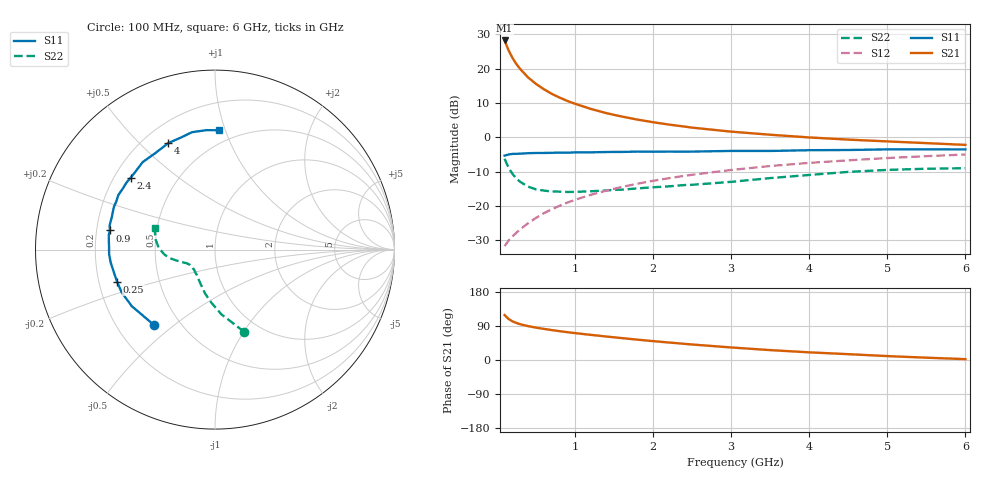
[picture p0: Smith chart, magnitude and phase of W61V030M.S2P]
! SIEMENS Small Signal Semiconductors
! BFR193W
! Si NPN RF Bipolar Junction Transistor in SOT323
! VCE = 1 V  IC = 30 mA
! Common Emitter S-Parameters:  September  1992
# GHz  S  MA  R  50
!  f  S11  S21  S12  S22
! GHz  MAG  ANG  MAG  ANG  MAG  ANG  MAG  ANG
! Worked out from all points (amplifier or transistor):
!   28 points, 100 MHz to 6 GHz, reference 50 ohm
!   highest |S21| = 28.3 dB at 100 MHz (marker M1)
!   |S21| within 3 dB of that: start of sweep to 153.5 MHz
!   unconditionally stable (mu >= 1): 511.2 MHz to 2.751 GHz
!   at 300 MHz: K = 0.88, MSG = 23.4 dB, |S12| = -26.8 dB
!   at 1.5 GHz: K = 1.05, MAG = 9.4 dB, |S12| = -15.0 dB
!   at 6 GHz: K = 0.96, MSG = 1.4 dB, |S12| = -5.0 dB
!   S11 on the Smith chart (normalised r, x): 100 MHz: 0.36, -0.43; 250 MHz: 0.28, -0.15; 900 MHz: 0.26, +0.08; 2.4 GHz: 0.27, +0.35; 4 GHz: 0.30, +0.61; 6 GHz: 0.40, +0.95
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0.1  0.5405 -128.7  25.86 118.6  0.0258 54.2  0.4863 -70.4
0.15  0.5606 -145.8  18.63 108.4  0.031 54.1  0.3615 -84.5
0.2  0.572 -155.4  14.44 102.0  0.0356 55.9  0.2939 -94.4
0.25  0.5742 -161.8  11.73 97.8  0.0404 58.3  0.2506 -102.7
0.3  0.5766 -166.4  9.899 94.4  0.0455 60.4  0.2239 -108.4
0.4  0.5858 -173.0  7.484 89.4  0.0557 63.9  0.1909 -118.3
0.5  0.5905 -177.7  6.028 85.5  0.0665 66.0  0.1741 -125.6
0.6  0.5906 178.3  5.049 82.2  0.0777 67.2  0.1671 -131.4
0.7  0.5937 175.2  4.328 79.0  0.0887 68.0  0.162 -135.4
0.8  0.5974 172.2  3.814 76.2  0.0997 68.3  0.1612 -138.8
0.9  0.5956 169.7  3.402 73.5  0.1112 68.5  0.1593 -141.5
1  0.6024 167.0  3.088 71.0  0.1222 68.3  0.1598 -143.6
1.2  0.6031 162.1  2.602 66.4  0.1443 67.6  0.1631 -148.2
1.4  0.6094 158.2  2.257 62.0  0.1664 66.6  0.1675 -150.9
1.6  0.6117 154.2  2.009 57.8  0.1885 65.4  0.1723 -153.5
2.2  0.6186 142.9  1.535 46.2  0.2527 61.0  0.1923 -158.2
2.4  0.6174 139.5  1.435 42.7  0.2737 59.3  0.2009 -159.8
3.5  0.6319 122.0  1.09 26.1  0.3808 49.1  0.2539 -168.9
4  0.6481 113.6  0.995 20.2  0.4232 44.4  0.2821 -174.2
4.5  0.6524 106.9  0.925 15.4  0.4607 39.9  0.3129 178.5
5.5  0.6672 94.1  0.822 6.1  0.5305 30.9  0.3477 164.1
6  0.665 88.3  0.775 2.3  0.5608 26.3  0.3535 159.7
